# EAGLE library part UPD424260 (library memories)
DRAM 256K x16 NEC Electronics Inc.
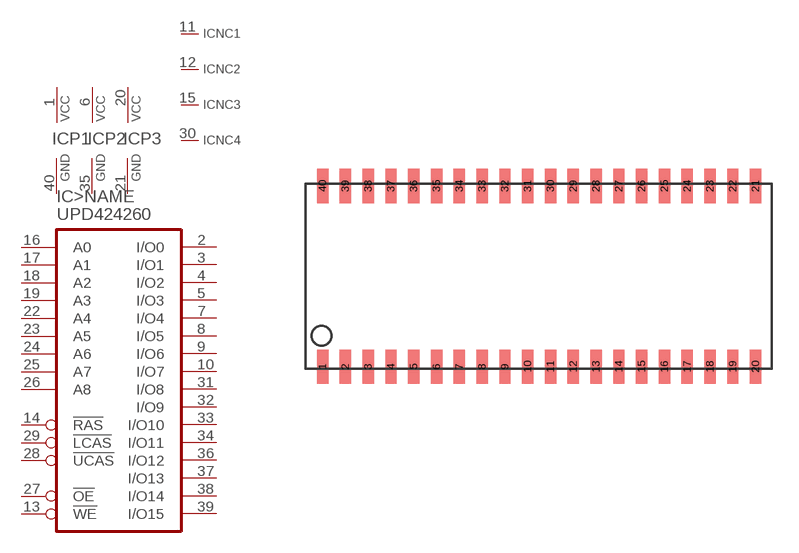
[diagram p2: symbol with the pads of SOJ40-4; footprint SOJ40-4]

Designator prefix IC; gates >NAME=DRAM256KX16 P1=PWRN P2=PWRN P3=PWRN NC1=NC NC2=NC NC3=NC NC4=NC

## UPD424260LE  [SOJ40-4]
1  P1:VCC  pwr
2  >NAME:I/O0  hiz
3  >NAME:I/O1  hiz
4  >NAME:I/O2  hiz
5  >NAME:I/O3  hiz
6  P2:VCC  pwr
7  >NAME:I/O4  hiz
8  >NAME:I/O5  hiz
9  >NAME:I/O6  hiz
10  >NAME:I/O7  hiz
11  NC1:NC  nc
12  NC2:NC  nc
13  >NAME:!WE  in
14  >NAME:!RAS  in
15  NC3:NC  nc
16  >NAME:A0  in
17  >NAME:A1  in
18  >NAME:A2  in
19  >NAME:A3  in
20  P3:VCC  pwr
21  P3:GND  pwr
22  >NAME:A4  in
23  >NAME:A5  in
24  >NAME:A6  in
25  >NAME:A7  in
26  >NAME:A8  in
27  >NAME:!OE  in
28  >NAME:!UCAS  in
29  >NAME:!LCAS  in
30  NC4:NC  nc
31  >NAME:I/O8  hiz
32  >NAME:I/O9  hiz
33  >NAME:I/O10  hiz
34  >NAME:I/O11  hiz
35  P2:GND  pwr
36  >NAME:I/O12  hiz
37  >NAME:I/O13  hiz
38  >NAME:I/O14  hiz
39  >NAME:I/O15  hiz
40  P1:GND  pwr

## Footprint SOJ40-4 (pad centres in mm)
Small Outline J-Bend
smd 0.635 x 1.905: 1 -10.16,-5.029; 2 -8.89,-5.029; 3 -7.62,-5.029; 4 -6.35,-5.029; 5 -5.08,-5.029; 6 -3.81,-5.029; 7 -2.54,-5.029; 8 -1.27,-5.029; 9 0,-5.029; 10 1.27,-5.029; 11 2.54,-5.029; 12 3.81,-5.029; 13 5.08,-5.029; 14 6.35,-5.029; 15 7.62,-5.029; 16 8.89,-5.029; 17 10.16,-5.029; 18 11.43,-5.029; 19 12.7,-5.029; 20 13.97,-5.029; 21 13.97,5.029; 22 12.7,5.029; 23 11.43,5.029; 24 10.16,5.029; 25 8.89,5.029; 26 7.62,5.029; 27 6.35,5.029; 28 5.08,5.029; 29 3.81,5.029; 30 2.54,5.029; 31 1.27,5.029; 32 0,5.029; 33 -1.27,5.029; 34 -2.54,5.029; 35 -3.81,5.029; 36 -5.08,5.029; 37 -6.35,5.029; 38 -7.62,5.029; 39 -8.89,5.029; 40 -10.16,5.029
